[IBIS Ver]   3.2
[File Name]   sprm192a.ibs
[File Rev]   0.1
[Date]   April 20, 2006
[Source]   File Originated at Texas Instruments
[Disclaimer]   Please be aware that in the absence of a written agreement
|   Texas Instruments(TI) assumes no liability for:
|   (1) The accuracy of the IBIS models provided to your company
|   (2) The proper functioning of these Models in your design
|   or for any resulting applications;or
|   (3) Infringement of patents,copyrights, or intellectual
|   property rights resulting from your use of these models.
|   TI provides IBIS Models as a service to our customers and
|   therefore reserves the right to limit distribution of the
|   Models.
[Copyright]   Property of Texas Instruments Incorporated.
|   Unauthorized reproduction and/or distribution is strictly
|   prohibited.
|   This product is protected under copyright law and trade
|   secret law as an unpublished work.
|   Created 1999,(C) Copyright 1999-2000,
|   Texas Instruments Incorporated., All Rights Reserved.
|   These commodities are under the U.S.
|   Government distribution license control.As such,they are not
|   to be re-exported without the prior approval of the U.S.
|   Department of Commerce.
[Component]   c6722_rfp
[Manufacturer]   Texas Instruments
[Package]
|Variable   Typ   Min   Max
R_pkg   2.350e-01   2.08059e-01 2.75017e-01
L_pkg   7.500e-09   6.68907e-09 8.78582e-09
C_pkg   1.750e-13   1.52265e-13 4.28149e-13
[Pin]   signal_name   model_name
2   AHCLKX0   BC3325BSHY
3   AMUTE0   BC3325BSHY
4   AMUTE1   BC3325BSHY
5   AHCLKX1   BC3325BSHY
7   ACLKX1   BC3325BSHY
9   ACLKR1   BC3325BSHY
11   AFSX1   BC3325BSHY
12   AFSR1   BC3325BSHY
14   RESET   IC33SHY
17   CLKIN   IC33SHY
19   TMS   IC33SHYPU
21   TRST   IC33SPD
28   TDI   IC33SHYPU
29   TDO   BC3325BSHYPU
32   EMU0   BC3325BSHYPU
34   EMU1   BC3325BSHYPU
35   TCK   IC33SHYPU
37   SDRAM_CAS   BC3325BSHY
38   EM_WE   BC3325BSHY
39   EM_WE_DQM[0]   BC3325BSHY
41   EM_D[7]   BC3325BSHY
43   EM_D[6]   BC3325BSHY
45   EM_D[5]   BC3325BSHY
46   EM_D[4]   BC3325BSHY
48   EM_D[3]   BC3325BSHY
49   EM_D[2]   BC3325BSHY
51   EM_D[1]   BC3325BSHY
52   EM_D[0]   BC3325BSHY
55   EM_D[15]   BC3325BSHY
56   EM_D[14]   BC3325BSHY
58   EM_D[13]   BC3325BSHY
59   EM_D[12]   BC3325BSHY
61   EM_D[11]   BC3325BSHY
63   EM_D[10]   BC3325BSHY
64   EM_D[9]   BC3325BSHY
66   EM_D[8]   BC3325BSHY
67   EM_WE_DQM[1]   BC3325BSHY
70   EM_CLK   BC3325BSHY
71   EM_SDCKE   BC3325BSHY
74   EM_A[11]   BC3325BSHY
75   EM_A[9]   BC3325BSHY
76   EM_A[8]   BC3325BSHY
79   EM_A[7]   BC3325BSHY
80   EM_A[6]   BC3325BSHY
83   EM_A[5]   BC3325BSHY
84   EM_A[4]   BC3325BSHY
86   EM_A[3]   BC3325BSHY
88   EM_A[2]   BC3325BSHY
89   EM_A[1]   BC3325BSHY
91   EM_A[0]   BC3325BSHY
93   EM_A[10]   BC3325BSHY
94   EM_BA[1]   BC3325BSHY
96   EM_BA[0]   BC3325BSHY
97   EM_CS[0]   BC3325BSHY
98   SDRAM_RAS   BC3325BSHY
100   EM_CS[1]   BC3325BSHY
102   EM_RNW   BC3325BSHY
104   EM_OE   BC3325BSHY
105   SPI0_ENA   BC3325BSHY
107   SPI0_SCS   BC3325BSHY
108   SPI0_SCLK   BC3325BSHY
110   SPI0_SIMO   BC3325BSHY
111   SPI0_SOMI   BC3325BSHY
113   AXR0[0]   BC3325BSHY
115   AXR0[1]   BC3325BSHY
116   AXR0[2]   BC3325BSHY
117   AXR0[3]   BC3325BSHY
119   AXR0[4]   BC3325BSHY
120   AXR0[5]   BC3325BSHY
121   AXR0[6]   BC3325BSHY
122   AXR0[7]   BC3325BSHY
126   AXR0[8]   BC3325BSHY
127   AXR0[9]   BC3325BSHY
130   AXR0[10]   BC3325BSHY
131   AXR0[11]   BC3325BSHY
134   AXR0[12]   BC3325BSHY
135   AXR0[13]   BC3325BSHY
137   AXR0[14]   BC3325BSHY
138   AXR0[15]   BC3325BSHY
139   ACLKR0   BC3325BSHY
141   AFSR0   BC3325BSHY
142   ACLKX0   BC3325BSHY
143   AHCLKR0   BC3325BSHY
144   AFSX0   BC3325BSHY
[Package Model]   RFP
[Define Package Model]  RFP
[Manufacturer]   Texas Instruments
[OEM]   Texas Instruments
[Description]   RFP
[Number Of Sections]  1
[Number Of Pins]  84
[Pin Numbers]
2   Len=0  R=0.2636374   L=8.46821e-09   C=2.45129e-13 /
3   Len=0  R=0.2594028   L=8.3026e-09   C=2.19192e-13 /
4   Len=0  R=0.2543633   L=8.13986e-09   C=2.06495e-13 /
5   Len=0  R=0.2525213   L=8.04522e-09   C=1.9916e-13 /
7   Len=0  R=0.2471067   L=7.83105e-09   C=1.84916e-13 /
9   Len=0  R=0.241245   L=7.61735e-09   C=1.69625e-13 /
11   Len=0  R=0.2385424   L=7.47596e-09   C=1.68152e-13 /
12   Len=0  R=0.2372647   L=7.4126e-09   C=1.6463e-13 /
14   Len=0  R=0.2363876   L=7.3287e-09   C=1.56952e-13 /
17   Len=0  R=0.2354599   L=7.24765e-09   C=1.63564e-13 /
19   Len=0  R=0.2347821   L=7.2093e-09   C=1.9307e-13 /
21   Len=0  R=0.2369866   L=7.29283e-09   C=1.54642e-13 /
28   Len=0  R=0.2491398   L=7.77243e-09   C=1.73292e-13 /
29   Len=0  R=0.2533927   L=7.90442e-09   C=1.74457e-13 /
32   Len=0  R=0.2638887   L=8.26982e-09   C=2.08266e-13 /
34   Len=0  R=0.2651394   L=8.41894e-09   C=2.21913e-13 /
35   Len=0  R=0.2697852   L=8.59367e-09   C=2.52411e-13 /
37   Len=0  R=0.2664518   L=8.70267e-09   C=4.26418e-13 /
38   Len=0  R=0.2575474   L=8.35761e-09   C=2.39647e-13 /
39   Len=0  R=0.2494428   L=8.117e-09   C=2.13396e-13 /
41   Len=0  R=0.2382013   L=7.77572e-09   C=1.93076e-13 /
43   Len=0  R=0.2305767   L=7.51895e-09   C=1.76458e-13 /
45   Len=0  R=0.221115   L=7.23565e-09   C=1.67275e-13 /
46   Len=0  R=0.2188196   L=7.14469e-09   C=1.65184e-13 /
48   Len=0  R=0.2180347   L=7.0477e-09   C=1.6289e-13 /
49   Len=0  R=0.2151583   L=6.95697e-09   C=1.55471e-13 /
51   Len=0  R=0.2107886   L=6.81487e-09   C=1.54911e-13 /
52   Len=0  R=0.2116574   L=6.80989e-09   C=1.58355e-13 /
55   Len=0  R=0.2089021   L=6.7165e-09   C=1.86494e-13 /
56   Len=0  R=0.208996   L=6.74414e-09   C=1.52265e-13 /
58   Len=0  R=0.2094584   L=6.78942e-09   C=1.56306e-13 /
59   Len=0  R=0.2097984   L=6.82276e-09   C=1.54623e-13 /
61   Len=0  R=0.2116496   L=6.92514e-09   C=1.53955e-13 /
63   Len=0  R=0.2161952   L=7.09379e-09   C=1.58923e-13 /
64   Len=0  R=0.2193198   L=7.20093e-09   C=1.63306e-13 /
66   Len=0  R=0.2275906   L=7.46109e-09   C=1.73346e-13 /
67   Len=0  R=0.2327107   L=7.61361e-09   C=1.79073e-13 /
70   Len=0  R=0.2528694   L=8.18324e-09   C=2.13205e-13 /
71   Len=0  R=0.2582552   L=8.37187e-09   C=2.41179e-13 /
74   Len=0  R=0.2750174   L=8.69481e-09   C=2.49089e-13 /
75   Len=0  R=0.2721328   L=8.5547e-09   C=2.25624e-13 /
76   Len=0  R=0.2678133   L=8.40566e-09   C=2.08111e-13 /
79   Len=0  R=0.2551967   L=7.99165e-09   C=1.86084e-13 /
80   Len=0  R=0.2536267   L=7.90927e-09   C=1.79605e-13 /
83   Len=0  R=0.2428024   L=7.56046e-09   C=1.66444e-13 /
84   Len=0  R=0.2438847   L=7.5423e-09   C=1.66714e-13 /
86   Len=0  R=0.2390976   L=7.3825e-09   C=1.56564e-13 /
88   Len=0  R=0.2387374   L=7.32709e-09   C=1.62827e-13 /
89   Len=0  R=0.2372399   L=7.28265e-09   C=1.64154e-13 /
91   Len=0  R=0.2359321   L=7.2321e-09   C=1.90614e-13 /
93   Len=0  R=0.2357966   L=7.26943e-09   C=1.58472e-13 /
94   Len=0  R=0.2363084   L=7.30102e-09   C=1.6084e-13 /
96   Len=0  R=0.236812   L=7.36846e-09   C=1.59235e-13 /
97   Len=0  R=0.2376596   L=7.41994e-09   C=1.58433e-13 /
98   Len=0  R=0.2390121   L=7.48472e-09   C=1.60595e-13 /
100  Len=0  R=0.2425698   L=7.64233e-09   C=1.71172e-13 /
102  Len=0  R=0.2476106   L=7.84039e-09   C=1.8381e-13 /
104  Len=0  R=0.2545687   L=8.08432e-09   C=1.91694e-13 /
105  Len=0  R=0.259766   L=8.24383e-09   C=2.03996e-13 /
107  Len=0  R=0.2643052   L=8.48167e-09   C=2.47617e-13 /
108  Len=0  R=0.2710598   L=8.78582e-09   C=4.28149e-13 /
110  Len=0  R=0.2597374   L=8.39131e-09   C=2.39273e-13 /
111  Len=0  R=0.2515128   L=8.1481e-09   C=2.11118e-13 /
113  Len=0  R=0.2379513   L=7.76152e-09   C=1.88342e-13 /
115  Len=0  R=0.2268967   L=7.43825e-09   C=1.74602e-13 /
116  Len=0  R=0.2224967   L=7.30147e-09   C=1.70133e-13 /
117  Len=0  R=0.218775   L=7.18035e-09   C=1.68331e-13 /
119  Len=0  R=0.2148724   L=7.01556e-09   C=1.58852e-13 /
120  Len=0  R=0.2124547   L=6.93e-09   C=1.55986e-13 /
121  Len=0  R=0.2107683   L=6.86207e-09   C=1.56865e-13 /
122  Len=0  R=0.2112976   L=6.8407e-09   C=1.59394e-13 /
126  Len=0  R=0.2080599   L=6.68907e-09   C=1.86574e-13 /
127  Len=0  R=0.2085121   L=6.6982e-09   C=1.91144e-13 /
130  Len=0  R=0.2102384   L=6.79342e-09   C=1.55268e-13 /
131  Len=0  R=0.2117284   L=6.84906e-09   C=1.52311e-13 /
134  Len=0  R=0.2174921   L=7.06592e-09   C=1.62247e-13 /
135  Len=0  R=0.2209152   L=7.17409e-09   C=1.65531e-13 /
137  Len=0  R=0.2263527   L=7.37542e-09   C=1.69015e-13 /
138  Len=0  R=0.2314906   L=7.52619e-09   C=1.74074e-13 /
139  Len=0  R=0.2373407   L=7.69311e-09   C=1.82893e-13 /
141  Len=0  R=0.245706   L=7.97023e-09   C=2.01348e-13 /
142  Len=0  R=0.2504994   L=8.12854e-09   C=2.11405e-13 /
143  Len=0  R=0.2582552   L=8.36327e-09   C=2.37195e-13 /
144  Len=0  R=0.2671298   L=8.70882e-09   C=4.22933e-13 /
[End_Package_Model]
[Component]   BC3325BSHY
[Manufacturer]   Texas Instruments
[Package]
|   typ   min   max
R_pkg   0   0   0
L_pkg   0   0   0
C_pkg   0   0   0
[Pin]   signal_name   model_name   R_pin   L_pin   C_pin
   1   Y   BC3325BSHY   0   0   0
[Component]   BC3325BSHYPU
[Manufacturer]   Texas Instruments
[Package]
|   typ   min   max
R_pkg   0   0   0
L_pkg   0   0   0
C_pkg   0   0   0
[Pin]   signal_name   model_name   R_pin   L_pin   C_pin
   1   Y   BC3325BSHYPU   0   0   0
[Component]   IC33SHY
[Manufacturer]   Texas Instruments
[Package]
|   typ   min   max
R_pkg   0   0   0
L_pkg   0   0   0
C_pkg   0   0   0
[Pin]   signal_name   model_name   R_pin   L_pin   C_pin
   1   A   IC33SHY   0   0   0
[Component]   IC33SHYPU
[Manufacturer]   Texas Instruments
[Package]
|   typ   min   max
R_pkg   0   0   0
L_pkg   0   0   0
C_pkg   0   0   0
[Pin]   signal_name   model_name   R_pin   L_pin   C_pin
   1   A   IC33SHYPU   0   0   0
[Component]   IC33SPD
[Manufacturer]   Texas Instruments
[Package]
|   typ   min   max
R_pkg   0   0   0
L_pkg   0   0   0
C_pkg   0   0   0
[Pin]   signal_name   model_name   R_pin   L_pin   C_pin
   1   A   IC33SPD   0   0   0
| Models and submodels in the file (5): BC3325BSHY (I/O), BC3325BSHYPU (I/O), IC33SHY (Input), IC33SHYPU (Input), IC33SPD (Input)
